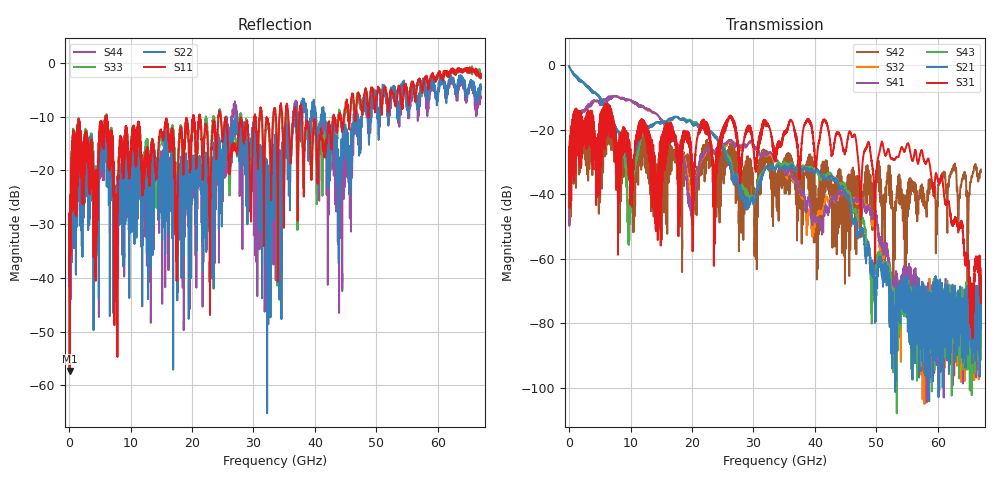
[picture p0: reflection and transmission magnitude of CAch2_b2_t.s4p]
!Agilent Technologies,N5247A,US51170199,A.09.90.13
!Agilent N5247A: A.09.90.13
!Date: Tuesday, October 23, 2018 13:01:32
!Correction: S11(Full 4 Port(1,2,3,4))
!S12(Full 4 Port(1,2,3,4))
!S13(Full 4 Port(1,2,3,4))
!S14(Full 4 Port(1,2,3,4))
!S21(Full 4 Port(1,2,3,4))
!S22(Full 4 Port(1,2,3,4))
!S23(Full 4 Port(1,2,3,4))
!S24(Full 4 Port(1,2,3,4))
!S31(Full 4 Port(1,2,3,4))
!S32(Full 4 Port(1,2,3,4))
!S33(Full 4 Port(1,2,3,4))
!S34(Full 4 Port(1,2,3,4))
!S41(Full 4 Port(1,2,3,4))
!S42(Full 4 Port(1,2,3,4))
!S43(Full 4 Port(1,2,3,4))
!S44(Full 4 Port(1,2,3,4))
!S4P File: Measurements: <S11,S12,S13,S14>,
!<S21,S22,S23,S24>,
!<S31,S32,S33,S34>,
!<S41,S42,S43,S44>:
# Hz S  dB  R 50
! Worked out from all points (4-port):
!   6701 points, 10 MHz to 67 GHz, reference 50 ohm
!   strongest paths, dB at 10 MHz, 16.76 GHz, 33.51 GHz, 50.25 GHz, 67 GHz:
!     S31: -33.2, -22.7, -27.3, -29.0, -70.6
!     S21: -0.4, -16.3, -32.2, -61.9, -78.8
!     S43: -0.4, -16.5, -32.1, -58.5, -75.0
!     S41: -48.5, -22.5, -29.8, -50.1, -75.0
!     S32: -48.4, -22.3, -29.9, -51.0, -68.1
!     S42: -33.4, -27.6, -33.0, -35.2, -32.4
!   lowest |S11| = -57.3 dB at 99.99 MHz (marker M1), VSWR 1.00, Z = 49.9 - j0.125 ohm
!   |S11| at or under -10 dB: start of sweep to 5.972 GHz; 6.104 GHz to 20.16 GHz (14.05 GHz wide, 107 % of centre); 24.68 GHz to 30.15 GHz (5.475 GHz wide, 20 % of centre)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
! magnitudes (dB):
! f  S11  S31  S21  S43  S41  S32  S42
! 10 MHz  -28.1  -33.2  -0.4  -0.4  -48.5  -48.4  -33.4
! 99.99 MHz  -57.3  -28.0  -0.8  -0.8  -42.4  -42.5  -28.4
! 7.739 GHz  -33.1  -38.7  -19.8  -19.9  -9.7  -9.6  -29.1
! 9.749 GHz  -18.3  -32.2  -31.6  -45.1  -10.7  -10.8  -29.1
! 42.42 GHz  -12.4  -23.0  -35.0  -33.3  -43.4  -41.7  -34.3
! 55.1 GHz  -6.0  -24.3  -70.4  -72.5  -64.9  -69.0  -45.5
! 67 GHz  -2.0  -70.6  -78.8  -75.0  -75.0  -68.1  -32.4
